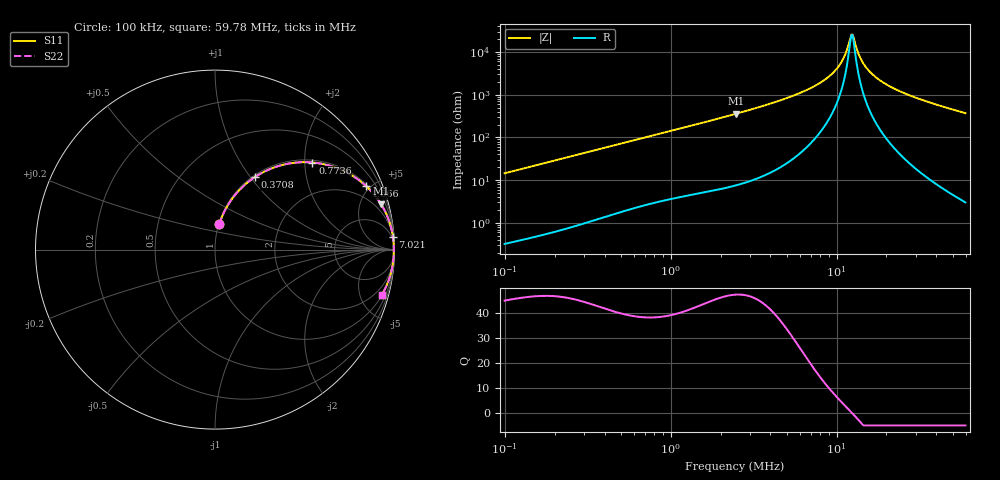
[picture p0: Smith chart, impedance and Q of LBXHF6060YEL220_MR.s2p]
! LBXHF6060YEL220_MR  S-PARAMETER MODEL  ( General Type )
! Model Generated by TAIYO YUDEN Corporation (http://www.ty-top.com)
! Version 1.0
! TAIYO YUDEN Control No. 200120NI43SB-FBB
! Copyright(c) 2020 TAIYO YUDEN CO.,LTD. All Rights Reserved.
! Product Description (link to TY-COMPAS)
! https://ds.yuden.co.jp/TYCOMPAS/or/detail?pn=LBXHF6060YEL220MMR&u=M
! Products Name : Inductors
! Characteristics :
!  Inductance : 22 uH , SRF(min) : 9.0 MHz , DC Resistance(max) : 0.132 Ohm
!  Rated Current : Saturation :2500 mA , Temp Rise : 1200 mA
!  Case Size : 6.0 x 6.0 / 0.236 x 0.236 [mm/inch] , Thickness : 4.5 / 0.177 [mm/inch]
!  (Conditions: Temperature = 25 degC , DC Bias Current/Voltage = 0A / 0V)
! External Node Assignments :
!  1  o---GGG---o  2
! GND o---------o GND
! Frequency Range : 0.1MHz  -  59.781294MHz  [ 402 STEP ]
# MHz S RI R 50
! Freq[MHz].  S11 Real  S11 Imag  S21 Real  S21 Imag  S12 Real  S12 Imag  S22 Real  S22 Imag
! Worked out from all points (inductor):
!   401 points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, 100 kHz to 59.78 MHz, reference 50 ohm
!   read as one part in series: L = 22.9 uH near 103.2 kHz
!   highest Q = 47.3 at 2.484 MHz (marker M1), where L = 22.9 uH
!   self-resonance near 12.28 MHz
!   S11 on the Smith chart (normalised r, x): 100 kHz: 1.01, +0.29; 370.8 kHz: 1.02, +1.06; 773.6 kHz: 1.06, +2.18; 1.666 MHz: 1.11, +4.71; 7.021 MHz: 2, +29; 59.78 MHz: 1.06, -7.38
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0.1  0.0235 0.1407  0.9765 -0.1407  0.9765 -0.1407  0.0235 0.1407
0.291793  0.1538 0.3497  0.8462 -0.3497  0.8462 -0.3497  0.1538 0.3497
0.370848  0.2239 0.4052  0.7761 -0.4052  0.7761 -0.4052  0.2239 0.4052
0.773572  0.5425 0.4853  0.4575 -0.4853  0.4575 -0.4853  0.5425 0.4853
0.851431  0.5878 0.4794  0.4122 -0.4794  0.4122 -0.4794  0.5878 0.4794
1.666053  0.8415 0.3541  0.1585 -0.3541  0.1585 -0.3541  0.8415 0.3541
2.484415  0.923 0.2562  0.077 -0.2562  0.077 -0.2562  0.923 0.2562
4.63382  0.9789 0.1306  0.0211 -0.1306  0.0211 -0.1306  0.9789 0.1306
7.021274  0.9917 0.0685  0.00831 -0.0685  0.00831 -0.0685  0.9917 0.0685
7.134398  0.992 0.0664  0.00803 -0.0664  0.00803 -0.0664  0.992 0.0664
8.642797  0.9945 0.0421  0.00552 -0.0421  0.00552 -0.0421  0.9945 0.0421
9.979919  0.9955 0.0249  0.00445 -0.0249  0.00445 -0.0249  0.9955 0.0249
10.98438  0.996 0.0138  0.00404 -0.0138  0.00404 -0.0138  0.996 0.0138
12.08994  0.9962 0.00281  0.00383 -0.00281  0.00383 -0.00281  0.9962 0.00281
12.48265  0.9962 -0.000848  0.0038 0.000848  0.0038 0.000848  0.9962 -0.000848
12.68377  0.9962 -0.00268  0.00379 0.00268  0.00379 0.00268  0.9962 -0.00268
13.96036  0.9961 -0.0137  0.00387 0.0137  0.00387 0.0137  0.9961 -0.0137
15.12181  0.9959 -0.023  0.0041 0.023  0.0041 0.023  0.9959 -0.023
17.18443  0.9952 -0.0382  0.00482 0.0382  0.00482 0.0382  0.9952 -0.0382
20.81767  0.9931 -0.0624  0.00695 0.0624  0.00695 0.0624  0.9931 -0.0624
32.05163  0.9813 -0.126  0.0187 0.126  0.0187 0.126  0.9813 -0.126
59.78129  0.9297 -0.2515  0.0703 0.2515  0.0703 0.2515  0.9297 -0.2515
